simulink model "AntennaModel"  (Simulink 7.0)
settings: Solver=ode45  StartTime=0.0  StopTime=20  MaxStep=0.01  RelTol=1e-3
libraries: cstblocks x4

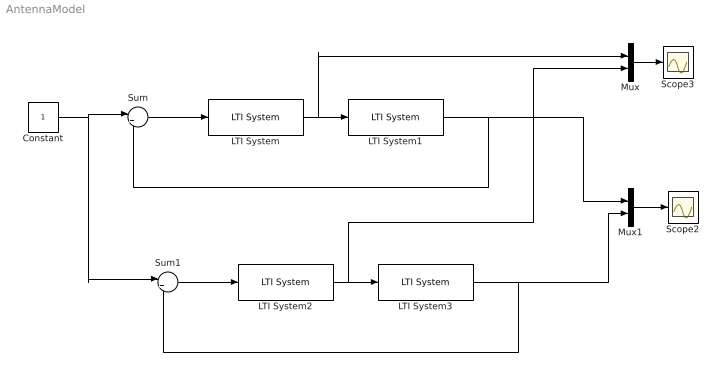
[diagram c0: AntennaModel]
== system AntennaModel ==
  Constant : Constant  OutDataType=sfix(16)  OutScaling=2^0
  LTI System : cstblocks/LTI System  SystemSampleTime=-1  sys=Cd  IC=[]
  LTI System1 : cstblocks/LTI System  SystemSampleTime=-1  sys=G  IC=[]
  LTI System2 : cstblocks/LTI System  SystemSampleTime=-1  sys=C  IC=[]
  LTI System3 : cstblocks/LTI System  SystemSampleTime=-1  sys=G  IC=[]
  Mux : Mux  Inputs=2
  Mux1 : Mux  Inputs=2
  Scope2 : Scope
  Scope3 : Scope
  Sum : Sum  Inputs=|+-  OutDataType=sfix(16)  OutScaling=2^0
  Sum1 : Sum  Inputs=|+-  OutDataType=sfix(16)  OutScaling=2^0
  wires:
  LTI System1/1 -> Sum/2, Mux1/1
  Sum/1 -> LTI System/1
  Constant/1 -> Sum/1, Sum1/1
  LTI System/1 -> LTI System1/1, Mux/1
  LTI System3/1 -> Sum1/2, Mux1/2
  Sum1/1 -> LTI System2/1
  LTI System2/1 -> LTI System3/1, Mux/2
  Mux1/1 -> Scope2/1
  Mux/1 -> Scope3/1
